FUNCTION "ManualUnloader" : VOID
TITLE =Manual unloader
VERSION : 0.1

BEGIN
NETWORK
TITLE =Inch forward unloader
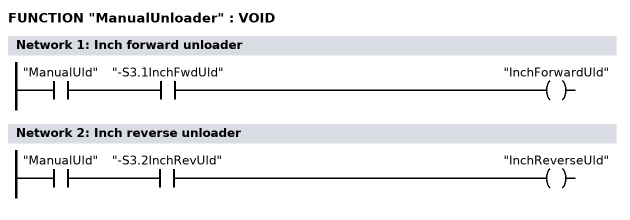
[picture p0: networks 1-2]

      A     "ManualUld";
      A     "-S3.1InchFwdUld";
      =     "InchForwardUld";
NETWORK
TITLE =Inch reverse unloader

      A     "ManualUld";
      A     "-S3.2InchRevUld";
      =     "InchReverseUld";
END_FUNCTION

